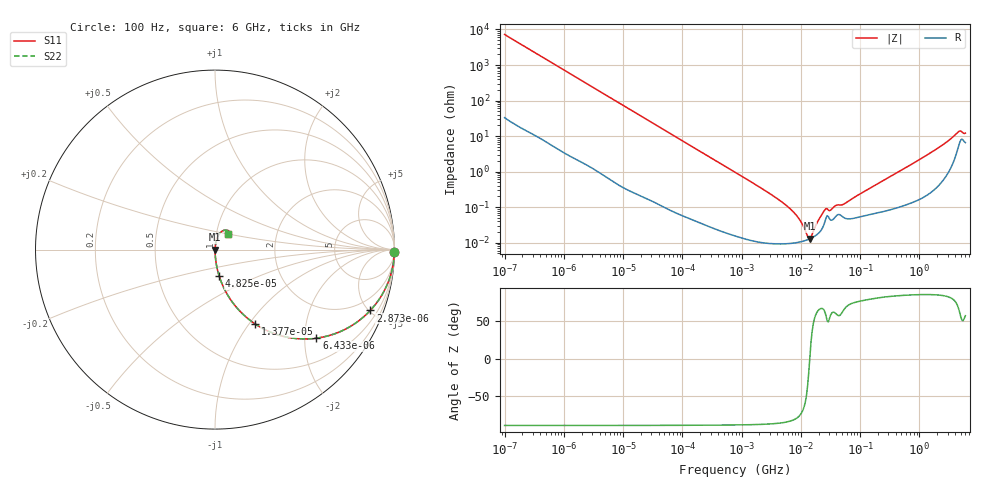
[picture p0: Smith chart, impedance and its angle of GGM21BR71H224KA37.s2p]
!Murata Part Number: GGM21BR71H224KA37
!These Parameters are Measured in Series Mode Connection
!Data Generated on Mar 13, 2026
!  o--ll--o
!Port1  Port2
!  o------o
!Operation Temp=25[degC], DC Bias Voltage=0[V]
!Freq. Start=100[Hz] Stop=6[GHz] 401[Steps]
# Hz S RI R 50
!Freq.(Hz) S11(Real) S11(Imag) S21(Real) S21(Imag) S12(Real) S12(Imag) S22(Real) S22(Imag)
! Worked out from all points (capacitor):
!   401 points, 100 Hz to 6 GHz, reference 50 ohm
!   read as one part in series: C = 220 nF near 109 Hz
!   lowest |Z| = 12.9 mohm at 14.22 MHz (marker M1)
!   series resonance near 14.15 MHz, so ESL is about 580 pH
!   S11 on the Smith chart (normalised r, x): 100 Hz: open; 2.873 kHz: 1.03, -5.09; 6.433 kHz: 1.01, -2.28; 13.77 kHz: 1.01, -1.07; 48.25 kHz: 1.00, -0.31; 6 GHz: 1.13, +0.20
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100  0.9997 -0.0138  0.000253 0.0138  0.000253 0.0138  0.9997 -0.0138
600  0.9929 -0.0818  0.00712 0.0818  0.00712 0.0818  0.9929 -0.0818
2008  0.9286 -0.255  0.0714 0.255  0.0714 0.255  0.9286 -0.255
2873  0.8649 -0.3392  0.1351 0.3392  0.1351 0.3392  0.8649 -0.3392
6433  0.5647 -0.4934  0.4353 0.4934  0.4353 0.4934  0.5647 -0.4934
13772  0.2226 -0.4135  0.7774 0.4135  0.7774 0.4135  0.2226 -0.4135
40335  0.0334 -0.1765  0.9666 0.1765  0.9666 0.1765  0.0334 -0.1765
48246  0.0238 -0.1491  0.9762 0.1491  0.9762 0.1491  0.0238 -0.1491
147774  0.00294 -0.05  0.9971 0.05  0.9971 0.05  0.00294 -0.05
774597  0.000247 -0.00962  0.9998 0.00962  0.9998 0.00962  0.000247 -0.00962
6075234  9.48e-05 -0.00101  0.9999 0.00101  0.9999 0.00101  9.48e-05 -0.00101
9090158  0.000102 -0.00049  0.9999 0.00049  0.9999 0.00049  0.000102 -0.00049
1.300572e7  0.000121 -9.14e-05  0.9999 9.14e-05  0.9999 9.14e-05  0.000121 -9.14e-05
1.422411e7  0.000128 5.5e-06  0.9999 -5.5e-06  0.9999 -5.5e-06  0.000128 5.5e-06
1.555665e7  0.000138 0.000104  0.9999 -0.000104  0.9999 -0.000104  0.000138 0.000104
1.946e7  0.000178 0.000364  0.9998 -0.000364  0.9998 -0.000364  0.000178 0.000364
2.545746e7  0.000384 0.000745  0.9996 -0.000745  0.9996 -0.000745  0.000384 0.000745
5.449875e7  0.000498 0.00114  0.9995 -0.00114  0.9995 -0.00114  0.000498 0.00114
3.124326e8  0.000875 0.0069  0.9991 -0.0069  0.9991 -0.0069  0.000875 0.0069
1.873145e9  0.00497 0.0409  0.995 -0.0409  0.995 -0.0409  0.00497 0.0409
4.385646e9  0.05 0.1076  0.95 -0.1076  0.95 -0.1076  0.05 0.1076
6e9  0.0699 0.0892  0.9301 -0.0892  0.9301 -0.0892  0.0699 0.0892
